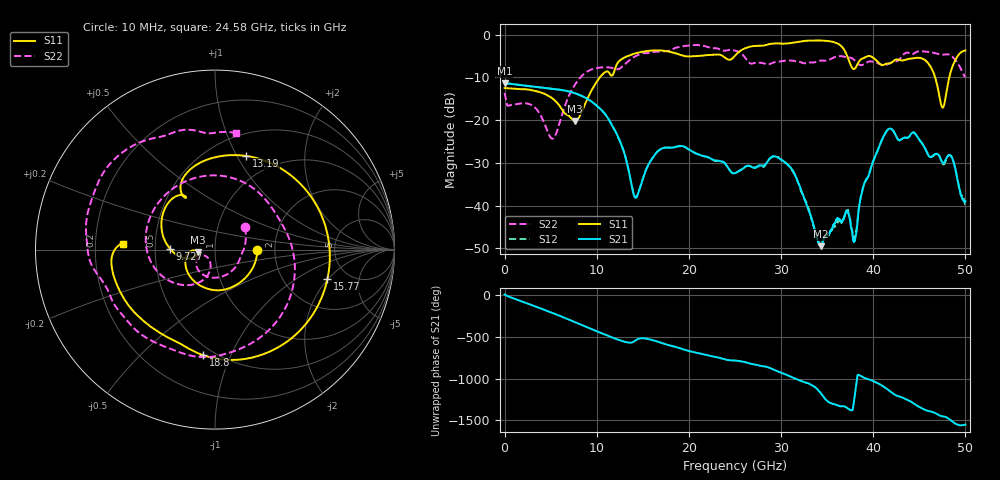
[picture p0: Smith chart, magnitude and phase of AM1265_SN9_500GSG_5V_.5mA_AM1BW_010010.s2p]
!Keysight Technologies,N5245B,MY58422270,A.16.20.02
!Date: Thursday, March 05, 2026 00:53:51
!Correction: S11(C  2-Port  )
!S21(C  2-Port  )
!S12(C  2-Port  )
!S22(C  2-Port  )
!S2P File: Measurements: S11, S21, S12, S22:
# Hz S  dB  R 50
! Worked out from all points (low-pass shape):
!   3201 points, 10 MHz to 50 GHz, reference 50 ohm
!   highest |S21| = -11.42 dB at 41.24 MHz (marker M1); lowest = -49.5 dB at 34.3 GHz (marker M2)
!   |S21| within 3 dB of the highest: start of sweep to 8.443 GHz
!   lowest |S11| = -20.2 dB at 7.665 GHz (marker M3), VSWR 1.22, Z = 41.2 - j1.16 ohm
!   |S11| at or under -10 dB: start of sweep to 10.35 GHz; 46.71 GHz to 48.25 GHz (1.538 GHz wide, 3.24 % of centre)
!   |S22| runs from -24.4 to -2.4 dB; largest |S21 - S12| = 0.0088
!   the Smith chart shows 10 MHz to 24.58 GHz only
!   S11 on the Smith chart (normalised r, x): 10 MHz: 1.62, -0.01; 9.727 GHz: 0.60, +0.01; 13.19 GHz: 0.73, +1.10; 15.77 GHz: 3.47, -1.98; 18.8 GHz: 0.44, -0.79; 24.58 GHz: 0.32, +0.03
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1e7  -12.51 -0.5  -11.42 5.1  -11.45 4.5  -13.66 36.6
4.124375e7  -12.52 -1.4  -11.42 3.5  -11.45 2.9  -14.00 31.6
5.212084e9  -14.96 -157.4  -12.71 144.2  -12.72 144.2  -24.36 -133.4
7.664719e9  -20.22 -171.8  -13.74 34.0  -13.73 34.1  -11.65 -130.9
8.352081e9  -18.25 -160.0  -14.33 2.2  -14.32 2.3  -9.77 -151.6
9.726806e9  -12.00 178.7  -16.15 -61.5  -16.13 -61.5  -7.96 160.1
1.141397e10  -9.16 120.0  -20.25 -138.9  -20.23 -138.9  -7.70 80.9
1.319486e10  -5.19 71.4  -29.28 155.0  -29.26 154.8  -6.66 -17.1
1.422591e10  -4.39 35.3  -38.17 176.8  -38.19 177.5  -5.05 -68.3
1.577247e10  -3.78 -14.8  -29.83 -172.2  -29.84 -172.1  -4.24 -121.4
1.667854e10  -3.69 -42.0  -27.21 159.2  -27.19 159.5  -4.02 -143.0
1.880312e10  -4.55 -96.4  -26.14 90.4  -26.18 90.5  -2.98 -179.9
2.458321e10  -5.80 176.7  -32.16 -63.3  -32.14 -62.7  -3.62 79.7
2.5005e10  -4.96 175.3  -32.43 -64.3  -32.41 -64.0  -3.75 70.2
2.951972e10  -2.06 96.4  -28.60 171.3  -28.45 170.7  -6.38 -18.2
3.334708e10  -1.40 35.6  -43.35 -0.7  -43.43 -2.8  -6.54 -132.7
3.430002e10  -1.39 19.1  -49.51 -94.2  -48.80 -94.6  -6.08 -153.7
3.80024e10  -7.97 -26.9  -48.28 -115.5  -47.45 100.6  -6.10 134.1
4.167354e10  -6.78 -54.5  -22.08 -59.9  -22.02 -59.8  -6.84 112.4
4.517284e10  -5.52 -101.6  -25.08 89.5  -25.11 89.7  -3.90 73.9
4.771921e10  -16.20 67.3  -29.94 -14.5  -30.24 -14.1  -4.66 40.6
5e10  -3.71 -71.1  -38.98 -111.9  -39.73 -106.5  -9.99 7.8
